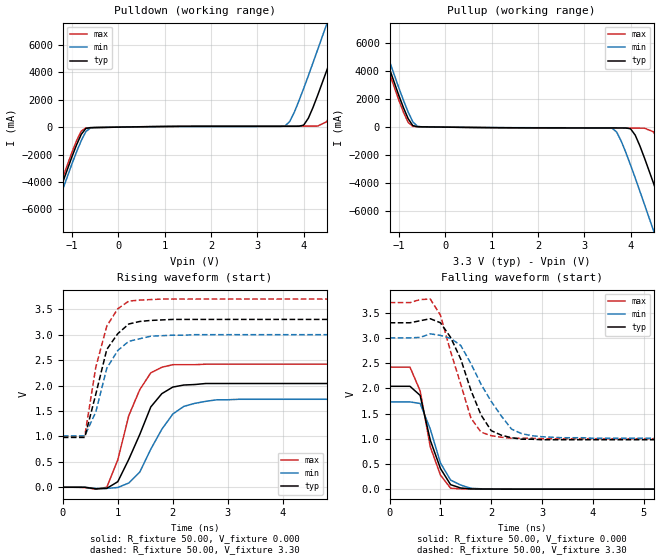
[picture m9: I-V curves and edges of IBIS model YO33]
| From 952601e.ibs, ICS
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|   Model YO33
[Model]   YO33
Model_type   Output
Polarity   Non-Inverting
C_comp   5.50pF   5.00pF   6.00pF
[Temperature Range]   27.00   70.00   0.000
[Voltage Range]   3.30V   3.00V   3.70V
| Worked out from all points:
|   slope of the pulldown table from 0 to 0.495 V, typ, clamps not added: 18 ohm
|   slope of the pullup table from 0 to 0.495 V, typ, clamps not added: 25.6 ohm
|   rising waveform, R_fixture 50.00, V_fixture 0.000: 20-80 % time 505ps typ, 542ps min, 430ps max; typ from 0 V to 2.04 V
|   rising waveform, R_fixture 50.00, V_fixture 3.30: 20-80 % time 372ps typ, 380ps min, 319ps max; typ from 0.98 V to 3.3 V
|   falling waveform, R_fixture 50.00, V_fixture 0.000: 20-80 % time 350ps typ, 378ps min, 325ps max; typ from 2.04 V to 0 V
|   falling waveform, R_fixture 50.00, V_fixture 3.30: 20-80 % time 536ps typ, 695ps min, 481ps max; typ from 3.3 V to 0.98 V
[Pulldown]
| voltage   I(typ)   I(min)   I(max)
-3.3V     -24.5A     -25.12A    -24.2A
-1.7V     -8.77A     -9.29A     -8.45A
-1.5V     -6.83A     -7.35A     -6.51A
-900mV    -1.27A     -1.78A     -970mA
-700mV    -92.33mA   -320mA     -53mA
3.6V      62.06mA    88.77mA    76.48mA
4V        150mA      2.83A      76.72mA
4.3V      2.31A      5.64A      77.26mA
4.5V      4.16A      7.55A      400mA
4.9V      8A         11.44A     3.83A
5.3V      11.9A      15.36A     7.68A
6.6V      24.75A     28.22A     20.49A
[Pullup]
| voltage   I(typ)   I(min)   I(max)
-3.3V     24.63A     25.13A     24.3A
-1.7V     8.89A      9.42A      8.55A
-1.5V     6.95A      7.49A      6.61A
-900mV    1.37A      1.9A       1.05A
-700mV    110mA      380mA      48.59mA
3.6V      -57.31mA   -72.21mA   -72.11mA
3.7V      -57.51mA   -350mA     -72.37mA
4V        -120mA     -2.71A     -73.07mA
4.5V      -4.04A     -7.42A     -340mA
4.9V      -7.88A     -11.31A    -3.73A
5.3V      -11.79A    -15.23A    -7.57A
6.6V      -24.65A    -28.1A     -20.38A
[Ramp]
| variable   typ   min   max
dV/dt_r   1.23/0.42n   1.04/0.53n   1.45/0.36n
dV/dt_f   1.39/0.50n   1.19/0.68n   1.62/0.40n
R_load = 50.00
[Rising Waveform]
R_fixture = 50.00
V_fixture = 0.000
V_fixture_min = 0.000
V_fixture_max = 0.000
| time   V(typ)   V(min)   V(max)
0s        79.81uV    57.94uV    260uV
800ps     -21.41mV   -21.71mV   420uV
1ns       110mV      -4.82mV    540mV
1.2ns     550mV      84.45mV    1.41V
1.4ns     1.04V      300mV      1.92V
1.6ns     1.58V      750mV      2.25V
2ns       1.97V      1.44V      2.41V
2.2ns     2.01V      1.59V      2.41V
2.8ns     2.04V      1.72V      2.42V
10ns      2.04V      1.73V      2.42V
[Rising Waveform]
R_fixture = 50.00
V_fixture = 3.30
V_fixture_min = 3.00
V_fixture_max = 3.70
| time   V(typ)   V(min)   V(max)
0s        980mV      1.01V      1V
400ps     980mV      1.01V      1.01V
600ps     1.83V      1.48V      2.36V
800ps     2.71V      2.34V      3.17V
1ns       3.02V      2.69V      3.51V
1.2ns     3.21V      2.87V      3.66V
1.4ns     3.26V      2.92V      3.68V
1.6ns     3.28V      2.97V      3.69V
2.4ns     3.3V       3V         3.7V
10ns      3.3V       3V         3.7V
[Falling Waveform]
R_fixture = 50.00
V_fixture = 0.000
V_fixture_min = 0.000
V_fixture_max = 0.000
| time   V(typ)   V(min)   V(max)
0s        2.04V      1.73V      2.42V
400ps     2.04V      1.73V      2.42V
600ps     1.86V      1.7V       1.95V
800ps     970mV      1.19V      840mV
1ns       410mV      520mV      280mV
1.2ns     88.56mV    180mV      19.04mV
1.4ns     22.96mV    80.63mV    6.22mV
1.6ns     5.06mV     17.25mV    3.31mV
2ns       1.83mV     2.57mV     1.17mV
10ns      780nV      -10.22uV   -4.65uV
[Falling Waveform]
R_fixture = 50.00
V_fixture = 3.30
V_fixture_min = 3.00
V_fixture_max = 3.70
| time   V(typ)   V(min)   V(max)
0s        3.3V       3V         3.7V
800ps     3.38V      3.08V      3.77V
1ns       3.3V       3.05V      3.45V
1.2ns     3.01V      2.99V      2.73V
1.4ns     2.58V      2.85V      2.08V
1.6ns     1.96V      2.49V      1.41V
2ns       1.16V      1.74V      1.06V
2.4ns     1.02V      1.19V      1.01V
3ns       980mV      1.04V      1V
10ns      980mV      1.01V      1V
